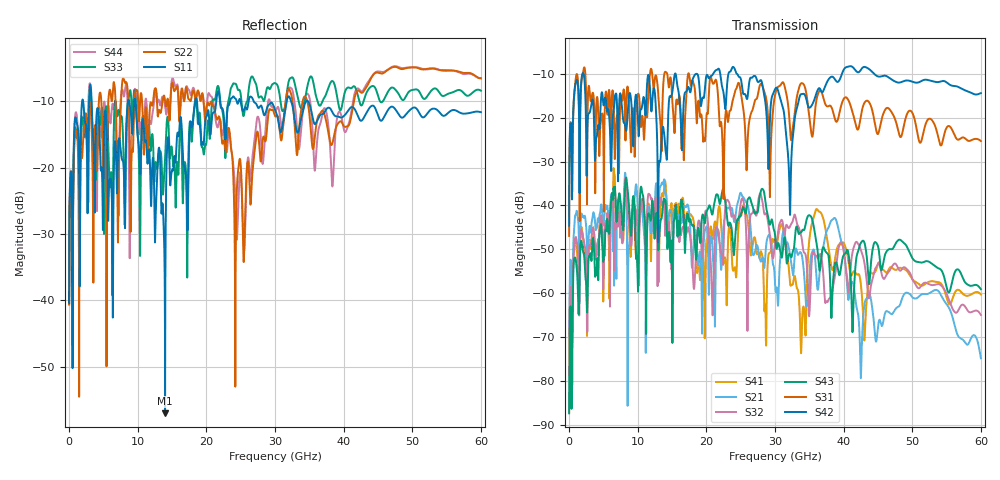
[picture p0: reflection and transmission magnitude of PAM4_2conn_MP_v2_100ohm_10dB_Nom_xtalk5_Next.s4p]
! Info: Touchstone file created by Circ.  Input file=FAB50GbE_2conn_Midplane_Examax_Topo2_v2_100ohm_10dB_Nom.circ
# Hz S RI R 50
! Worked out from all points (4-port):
!   6000 points, 10 MHz to 60 GHz, reference 50 ohm
!   strongest paths, dB at 10 MHz, 15.01 GHz, 30.01 GHz, 45.01 GHz, 60 GHz:
!     S42: -44.6, -14.5, -13.5, -10.6, -14.4
!     S31: -47.0, -15.3, -14.9, -23.7, -25.3
!     S43: -87.4, -52.6, -46.7, -49.3, -59.1
!     S32: -69.8, -56.7, -48.6, -53.3, -65.0
!     S21: -69.3, -43.7, -57.9, -67.7, -74.9
!     S41: -87.2, -41.5, -47.8, -53.3, -60.3
!   lowest |S11| = -57.0 dB at 13.99 GHz (marker M1), VSWR 1.00, Z = 50.1 + j0.00373 ohm
!   |S11| at or under -10 dB: 3.29 GHz to 8.582 GHz (5.292 GHz wide, 89.1 % of centre); 9.683 GHz to 18.39 GHz (8.71 GHz wide, 62 % of centre); 34.83 GHz to end of sweep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
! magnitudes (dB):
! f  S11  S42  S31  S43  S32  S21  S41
! 10 MHz  -40.4  -44.6  -47.0  -87.4  -69.8  -69.3  -87.2
! 2.02 GHz  -9.8  -9.8  -9.9  -50.3  -46.9  -42.4  -47.2
! 13.99 GHz  -57.0  -26.4  -9.6  -39.0  -46.4  -36.8  -34.4
! 33.86 GHz  -12.4  -14.6  -12.1  -46.1  -47.2  -51.1  -71.7
! 36.13 GHz  -13.0  -14.0  -15.3  -49.2  -51.8  -58.3  -40.9
! 43.03 GHz  -12.3  -8.4  -16.6  -48.5  -53.1  -62.7  -70.8
! 60 GHz  -11.6  -14.4  -25.3  -59.1  -65.0  -74.9  -60.3
